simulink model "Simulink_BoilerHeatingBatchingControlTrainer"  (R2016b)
settings: Solver=VariableStepAuto  StartTime=0.0  StopTime=10000  RelTol=1e-3
libraries: simulink x28, sldrtlib x1
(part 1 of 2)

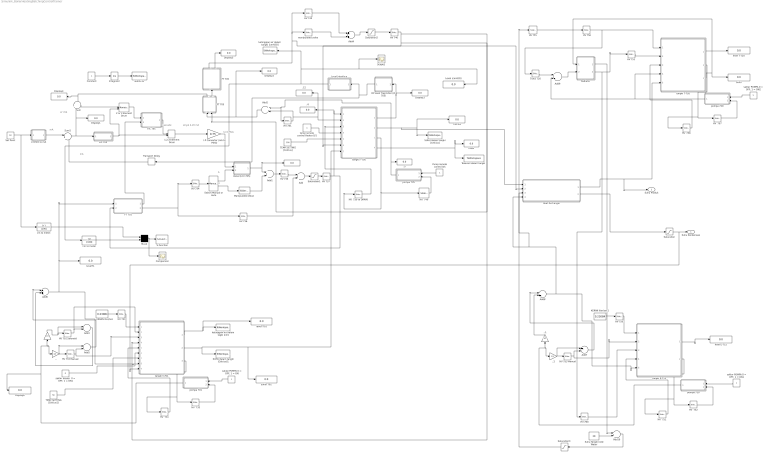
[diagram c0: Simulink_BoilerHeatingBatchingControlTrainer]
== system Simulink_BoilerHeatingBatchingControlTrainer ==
  note: Cascade
  note: 3-15 PSIG
  note: sinyal 4-20 mA
  note: mA
  note: mA
  note: A
  note: M
  note: LY 705
  ,. : Gain  RequirementInfo={} %GIDa_bc6fd614_1e62_4264_bb40_c7e61a15a363  Gain=1/2
  ,.1 : Gain  RequirementInfo={} %GIDa_cd3a2171_fe69_4d4d_90e5_3d5dc6404d7a  Gain=1/2
  .{,4..5,12} (4 alike) : Display
  .. : Gain  RequirementInfo={} %GIDa_859532f5_c8c5_4781_ad2a_2db76b1b0162  Gain=1/2
  ..1 : Gain  RequirementInfo={} %GIDa_722c5080_becd_473d_ad40_ed0b84a7ea39  Gain=1/2
  1,2,3 Element Drum : ManualSwitch  RequirementInfo={} %GIDa_e58d0757_014f_44f7_80c0_e7d97992c8d3
  2 or 3 Element Drum : ManualSwitch  RequirementInfo={} %GIDa_d69926c1_c1c0_413a_8fbd_7b981b4ad26d
  Add : Sum  RequirementInfo={} %GIDa_c8390c13_8fd0_46df_8b58_13085c3a574c
  Add1 : Sum  RequirementInfo={} %GIDa_43a3cd99_9539_4bf4_aa38_f64441418061
  Add10 : Sum
  Add2 : Sum  RequirementInfo={} %GIDa_35422669_7b0e_4bcd_b576_fa91f67b7c5f  Inputs=+-
  Add3 : Sum  RequirementInfo={} %GIDa_245dbbd9_2a0c_48cd_a41a_d83b265a6bdd  Inputs=+-
  Add4 : Sum  RequirementInfo={} %GIDa_1ca55e4e_7342_4df2_928e_79c2ac039fe9
  Add5 : Sum  RequirementInfo={} %GIDa_0dae67ae_8a33_45ca_89f9_5b09ff576389  Inputs=+-
  Add6 : Sum  RequirementInfo={} %GIDa_dee49598_737e_4bad_9513_14ba838757e0
  Add7 : Sum  RequirementInfo={} %GIDa_2ce0eeb6_1b8d_4e7c_881e_5b71408a7b6b  Inputs=+-
  Add8 : Sum  RequirementInfo={} %GIDa_35156967_a8ad_416d_ba36_a8f07401a50b
  Add9 : Sum
  Celcius : Display
  Comparison : Scope
  Constant : Constant  RequirementInfo={} %GIDa_0a77b0a1_350e_440f_9ee6_370cb4b1a8c2
  DP level Trasmitter (LT 705) : Subsystem  RequirementInfo={} %GIDa_fc1ec414_0db0_44f5_8f4f_154f58e86ad4
  Display{1..6} (6 alike) : Display
  FIC 701 : Subsystem  RequirementInfo={} %GIDa_2fdcdd1a_f8c8_4faf_bf04_b6ec306174f3
  FT 701 : Subsystem  RequirementInfo={} %GIDa_a0f6cfab_fe60_4a23_9956_c3a14955b270
  FT 705 : Subsystem  RequirementInfo={} %GIDa_2a8cb2f5_cffc_4b5e_9a3b_0ab803570460
  "HV  731 " : simulink/Math Operations/Slider Gain  low=0  gain=0  high=1
  HV  732 : simulink/Math Operations/Slider Gain  low=0  gain=1  high=1
  "HV  739 to DRAIN " : simulink/Math Operations/Slider Gain  low=0  gain=0  high=1
  "HV  740 " : simulink/Math Operations/Slider Gain  low=0  gain=1  high=1
  "HV  751 " : simulink/Math Operations/Slider Gain  low=0  gain=0  high=1
  HV  752 : simulink/Math Operations/Slider Gain  low=0  gain=1  high=1
  HV  757 : simulink/Math Operations/Slider Gain  low=0  gain=0  high=1
  HV  758 : simulink/Math Operations/Slider Gain  low=0  gain=0  high=1
  HV 701 Selenoid : simulink/Math Operations/Slider Gain  low=0  gain=0  high=1
  HV {730,735,750,756} (4 alike) : simulink/Math Operations/Slider Gain  low=0  gain=1  high=1
  HV 733 Manual : simulink/Math Operations/Slider Gain  low=0  gain=0  high=1
  "HV 734 " : simulink/Math Operations/Slider Gain  low=0  gain=1  high=1
  "HV 736 " : simulink/Math Operations/Slider Gain  low=0  gain=0  high=1
  "HV 737 " : simulink/Math Operations/Slider Gain  low=0  gain=1  high=1
  "HV 741 " : simulink/Math Operations/Slider Gain  low=0  gain=0  high=1
  HV 745 : simulink/Math Operations/Slider Gain  low=0  gain=0  high=1
  "HV 746 " : simulink/Math Operations/Slider Gain  low=0  gain=0.42086  high=1
  HV 751 : simulink/Math Operations/Slider Gain  low=0  gain=0  high=1
  HV 753 Manual : simulink/Math Operations/Slider Gain  low=0  gain=0  high=1
  "HV 755 " : simulink/Math Operations/Slider Gain  low=0  gain=1  high=1
  HV 760 : simulink/Math Operations/Slider Gain  low=0  gain=0  high=1
  Heat Exchanger : Subsystem
  I-P Converter (mA to PSIG) : Gain  RequirementInfo={} %GIDa_94b4f86c_9518_4108_a00c_4c2df90be3c9  Gain=0.75
  Integrator : Integrator  RequirementInfo={} %GIDa_4e981432_c823_455d_abdb_dc0f96a2a81a
  KERAN liter/sec : Constant  RequirementInfo={} %GIDa_cd72188c_dece_4be4_a14c_18aa689ca944  Value=0.23084
  KERAN liter/sec1 : Constant  RequirementInfo={} %GIDa_347f128a_a42e_4583_8b7f_c9f9fa14a285  Value=0.23084
  LIC 705 : Subsystem  RequirementInfo={} %GIDa_6249f34d_5a8b_41d9_ab20_0f82bded8f5b
  Level (cmH2O) : Display
  Level interface : Subsystem
  Manipulated Value : simulink/Math Operations/Slider Gain  low=0  gain=0  high=1
  Mux2 : Mux  RequirementInfo={} %GIDa_29235980_f912_414a_b16b_746e8be0c17d  Inputs=2
  PT 705 : Subsystem  RequirementInfo={} %GIDa_035bf6b7_6e08_480d_9a76_687a544ea6fb
  Pump remote control 0/1 : Constant  RequirementInfo={} %GIDa_9d76e44e_0bfb_4235_a62c_3277d40e00dd
  Radiator : Subsystem
  S-Function : S-Function  RequirementInfo={} %GIDa_3457ab31_c587_4ad5_a8ae_f74312ab7fb9  FunctionName=animtank  Parameters=1  SFunctionDeploymentMode=off  EnableBusSupport=off
  SUHU dalam tangki [Celcius] : ToWorkspace  VariableName=suhuF705  SampleTime=-1
  SUHU dalam tangki [Celcius]1 : ToWorkspace  VariableName=suhuT701  SampleTime=-1
  Saturation : Saturate  UpperLimit=5  LowerLimit=-9999999999999999999999  LinearizeAsGain=off
  Saturation1 : Saturate  RequirementInfo={} %GIDa_92280b64_3dca_498a_8f97_4b922c6ffe72  UpperLimit=1  LowerLimit=-99999999999999999999  LinearizeAsGain=off  ZeroCross=off
  Saturation2 : Saturate  RequirementInfo={} %GIDa_c6f00ae1_779b_49a9_846a_d92e31b6929e  UpperLimit=1  LowerLimit=-99999999999999999999  LinearizeAsGain=off  ZeroCross=off
  Saturation3 : Saturate  UpperLimit=28  LowerLimit=-9999999999999999  LinearizeAsGain=off
  Scope1 : Scope
  Set Point : Constant  Value=50
  Suhu : Display
  Suhu Tangki Cold Water : Constant  Value=28
  Sum : Sum  RequirementInfo={} %GIDa_2344363e_6328_49b0_a0c7_49a7caf909fe
  Sum1 : Sum  RequirementInfo={} %GIDa_c9939160_f8c3_468b_92a8_c76b635c367b  Inputs=|+-
  Switch Manual or Auto : simulink/Signal Routing/Manual Variant Sink  NumChoices=2  OverrideUsingVariant=V_1
  TEMP SETTING [Celcius] : Constant  RequirementInfo={} %GIDa_c1241bea_a72e_4e3d_bd4c_e18ce5dfffc9  Value=100
  TEMP SETTING [Celcius]1 : Constant  RequirementInfo={} %GIDa_1ee9e53c_fcbf_4bbe_a5b7_429d3d89aa33  Value=58
  TV/LV 720 : simulink/Math Operations/Slider Gain  low=0  gain=0  high=1
  "Tekanan dalam tangki " : ToWorkspace  VariableName=PressureF705  SampleTime=-1
  Transport Delay : TransportDelay
  Valve (LCV 705) : Subsystem  RequirementInfo={} %GIDa_cd02d2c4_9346_4b3f_af1b_c75ea5c89284
  cm to meter : TransferFcn  RequirementInfo={} %GIDa_bbce1113_4bf0_4329_b7d1_9b94b9680a34  Denominator=[100]
  cm to meter. : TransferFcn  RequirementInfo={} %GIDa_b4884718_8c5b_4fb0_8dff_b77bebcfc2f4  Denominator=[100]
  cmH2O to mA : Subsystem  RequirementInfo={} %GIDa_14021b81_10be_46ab_9522_3e35a22257df
  ketinggian air dalam tagki [cm] : ToWorkspace  VariableName=levelT701  SampleTime=-1
  ketinggian air dalam tangki [cmH2O] : ToWorkspace  VariableName=levelF705  SampleTime=-1
  level E-715 : Display
  level T-720 : Display
  levelT1 : Display
  levelT701 : Display
  manipulated valve : simulink/Math Operations/Slider Gain  low=0  gain=0.4  high=1
  mbar : Display
  pompa 701 : Subsystem  RequirementInfo={} %GIDa_f7b4c754_61d7_4523_a81d_5256af5e1442
  pompa 705 : Subsystem  RequirementInfo={} %GIDa_02e24820_9fe5_4fd9_b259_287392cabf84
  pompa 710 : Subsystem  RequirementInfo={} %GIDa_b40a5599_de7f_4543_949f_3323316adce9
  pompa 720 : Subsystem  RequirementInfo={} %GIDa_f39004c0_b4ae_4207_b1f8_c634ffc86dde
  "saklar heater  0 = OFF, 1 = ON1" : Constant  RequirementInfo={} %GIDa_29de96b5_5b8c_45ee_9680_99e645fe6211  Value=0
  "saklar POMPA 0 = OFF, 1 = ON" : Constant  RequirementInfo={} %GIDa_a2852ddb_fd6c_410b_b77d_b834fbe16be1
  "saklar POMPA 0 = OFF, 1 = ON1" : Constant  RequirementInfo={} %GIDa_d849ad1c_b491_4c30_8654_50d8025a813b
  "saklar POMPA 0 = OFF, 1 = ON2" : Constant  RequirementInfo={} %GIDa_87c96371_1090_42d7_9fd6_9dd4cd23a96a
  suhuT701 : Display
  tangki E-715 : Subsystem  RequirementInfo={} %GIDa_7bb4fadf_321c_4784_a602_bcf40fa0e2b0
  tangki F-705 : Subsystem  RequirementInfo={} %GIDa_ed91acdd_745b_4032_84c5_2be48a41ff32
  tangki T-701 : Subsystem  RequirementInfo={} %GIDa_4afd4461_0754_42e6_9c77_3d28637661d7
  tangki T-720 : Subsystem  RequirementInfo={} %GIDa_6bab6ea5_4044_4b9e_bbaf_a20bbf9bb028
  temp remote control Heater 0/1 : Constant  RequirementInfo={} %GIDa_5fa8f3d8_80e1_44eb_9f78_5bcca4947130
  waktu-ta' : ToWorkspace  VariableName=time  SampleTime=-1
  Suhu Kondensasi : Outport
  Suhu Produk : Outport  Port=2
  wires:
  Constant/1 -> Integrator/1
  tangki F-705/3(flow out [Liter/sec]) -> "HV  739 to DRAIN "/1, "HV  740 "/1
  "HV  739 to DRAIN "/1 -> tangki F-705/3(In6)
  "HV 736 "/1 -> Add/2
  HV 735/1 -> Add/1
  TEMP SETTING [Celcius]/1 -> tangki F-705/5(setting)
  FT 705/1(Out1) -> Display4/1, Sum/1
  FIC 701/1(Control) -> 1,2,3 Element Drum/1
  Add/1 -> Saturation1/1
  Mux2/1 -> S-Function/1, Comparison/1
  Pump remote control 0/1/1 -> pompa 705/1(saklar remote)
  Integrator/1 -> waktu-ta'/1
  FT 705/2("Out2 ") -> PT 705/1("In ")
  "HV 741 "/1 -> Add2/2, .12/1, tangki F-705/2(In2)
  "HV 734 "/1 -> Switch Manual or Auto/1
  Switch Manual or Auto/2 -> Manipulated Value/1
  Manipulated Value/1 -> Add1/2
  Add1/1 -> HV 735/1
  FT 701/2(Out2) -> "HV 734 "/1, "HV 736 "/1
  pompa 705/1(Out1) -> .5/1, Add2/1, "HV 741 "/1
  tangki F-705/4(Pressure (Pa)) -> mbar/1, "Tekanan dalam tangki "/1
  cm to meter/1 -> Mux2/2
  cm to meter./1 -> Mux2/1
  Set Point/1 -> cm to meter./1, cmH2O to mA/1(In1)
  cmH2O to mA/1(Out1) -> Sum1/1
  Switch Manual or Auto/1 -> Valve (LCV 705)/2(In2)
  I-P Converter (mA to PSIG)/1 -> Valve (LCV 705)/1(In1)
  Valve (LCV 705)/1(Out1) -> ./1, Add1/1
  LIC 705/1(Control) -> 2 or 3 Element Drum/2, 1,2,3 Element Drum/2
  temp remote control Heater 0/1/1 -> tangki F-705/4(remote on/off)
  Level interface/1(Out1) -> ketinggian air dalam tangki [cmH2O]/1, Scope1/1, Level (cmH2O)/1, cm to meter/1
  PT 705/2(Pressure Flow) -> Display5/1
  "HV  740 "/1 -> pompa 705/2(In2)
  Add6/1 -> levelT1/1, FT 701/1(In), tangki T-701/8(In7)
  Saturation2/1 -> "HV 746 "/1
  Add4/1 -> Saturation2/1
  manipulated valve/1 -> Add4/2
  HV 745/1 -> Add4/1
  "HV 746 "/1 -> tangki T-701/4(In4), FT 705/2(Valve), tangki F-705/6(In3)
  DP level Trasmitter (LT 705)/1(Out1) -> Transport Delay/1, Level interface/1(In1)
  Add2/1 -> FT 705/1(In), Display2/1
  Transport Delay/1 -> Sum1/2
  tangki F-705/1(level [cm]) -> Display3/1, DP level Trasmitter (LT 705)/1(In1)
  2 or 3 Element Drum/1 -> FIC 701/1(Set Point)
  Saturation1/1 -> "HV 737 "/1
  1,2,3 Element Drum/1 -> I-P Converter (mA to PSIG)/1
  Sum/1 -> 2 or 3 Element Drum/1
  Sum1/1 -> Display1/1, Sum/2, LIC 705/1(error)
  "HV 737 "/1 -> FT 701/2(valve), .4/1, tangki F-705/1(In1)
  FT 701/1(Out1) -> FIC 701/2(flow in)
  tangki T-701/1(level [cm]) -> ketinggian air dalam tagki [cm]/1, levelT701/1
  HV 730/1 -> tangki T-701/1(In1)
  KERAN liter/sec/1 -> HV 730/1
  pompa 701/1(Out1) -> ,./1, ../1, Display6/1
  "saklar POMPA 0 = OFF, 1 = ON"/1 -> pompa 701/1(saklar remote)
  tangki T-701/3(debit out (Liter/sec)) -> "HV  731 "/1, HV  732/1
  "HV  731 "/1 -> tangki T-701/5(In6)
  TEMP SETTING [Celcius]1/1 -> tangki T-701/7(setting)
  HV 733 Manual/1 -> tangki T-701/3(In3), Add5/2
  HV 701 Selenoid/1 -> tangki T-701/2(In2), Add3/2
  Add3/1 -> Add6/2
  Add5/1 -> Add6/1
  ../1 -> Add3/1, HV 701 Selenoid/1
  ,./1 -> Add5/1, HV 733 Manual/1
  HV  732/1 -> pompa 701/2(In2)
  "saklar heater  0 = OFF, 1 = ON1"/1 -> tangki T-701/6(remote on/off)
  Saturation/1 -> tangki T-701/9(Suhu Kondensasi), Suhu Kondensasi/1
  Heat Exchanger/1(Out1) -> tangki T-720/5(Suhu T-720), Suhu Produk/1
  Heat Exchanger/2(Out2) -> Saturation/1
  tangki F-705/2(suhu [Celcius]) -> Heat Exchanger/1(In1), Celcius/1, SUHU dalam tangki [Celcius]/1
  PT 705/1(Out1) -> Heat Exchanger/2(In2), HV 745/1, manipulated valve/1
  Add8/1 -> "HV 755 "/1, Heat Exchanger/4(In4), tangki E-715/5(In7)
  tangki T-701/2(suhu [Celcius]) -> tangki F-705/7(Suhu dari Heat Exchager), suhuT701/1, SUHU dalam tangki [Celcius]1/1
  tangki E-715/1(level [cm]) -> level E-715/1
  HV 750/1 -> tangki E-715/1(In1)
  KERAN liter/sec1/1 -> HV 750/1
  HV 760/1 -> tangki E-715/3(In4)
  pompa 710/1(Out1) -> ,.1/1, ..1/1
  "saklar POMPA 0 = OFF, 1 = ON1"/1 -> pompa 710/1(saklar remote)
  tangki E-715/2(debit out (Liter/sec)) -> "HV  751 "/1, HV  752/1
  "HV  751 "/1 -> tangki E-715/4(In6)
  HV 753 Manual/1 -> tangki E-715/2(In3), Add7/2
  ..1/1 -> Add8/2
  Add7/1 -> Add8/1
  ,.1/1 -> Add7/1, HV 753 Manual/1
  HV  752/1 -> pompa 710/2(In2)
  Radiator/2(Out2) -> HV 760/1, HV 751/1
  tangki T-720/1(level [cm]) -> level T-720/1
  "HV 755 "/1 -> HV 756/1
  "saklar POMPA 0 = OFF, 1 = ON2"/1 -> pompa 720/1(saklar remote)
  tangki T-720/2(debit out (Liter/sec)) -> HV  758/1, HV  757/1
  HV  758/1 -> tangki T-720/3(In6)
  HV  757/1 -> pompa 720/2(In2)
  HV 756/1 -> TV/LV 720/1, tangki T-720/1(In3)
  HV 751/1 -> tangki T-720/2(In4)
  TV/LV 720/1 -> Add9/1
  Add9/1 -> Radiator/2(In2)
  pompa 720/1(Out1) -> tangki T-720/4(In7), Add9/2
  tangki T-720/3(Suhu. T-720) -> Radiator/1(In1), Suhu/1
  Suhu Tangki Cold Water/1 -> Add10/2
  Add10/1 -> Saturation3/1
  Radiator/1(Out1) -> Add10/1
  Saturation3/1 -> Heat Exchanger/3(In3)

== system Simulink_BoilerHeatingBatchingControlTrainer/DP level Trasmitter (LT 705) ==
  note: P
  note: Tekanan hidrostatis P = p g h dimana P = Tekanan hidrostatis (N/m^2) g = percepatan gravitasi (m/s^2) p = massa jenis air (kg/m^3) h = level fluida
  note: mA
  In1 : Inport  RequirementInfo={} %GIDa_65631801_4d77_4024_98a1_8120f602e0b4
  Bias : Bias  RequirementInfo={} %GIDa_f33fa9ee_ffc2_4756_a0a9_dfedda8f7d97  Bias=4
  DP Level Transmitter Transfer Function : TransferFcn  RequirementInfo={} %GIDa_e8153e25_1b53_45ed_b90f_907755ff59fb  Numerator=[0.0016]  Denominator=[2 1]
  Saturation : Saturate  RequirementInfo={} %GIDa_8eb5f573_8386_419d_8ff5_e8c857dd8568  UpperLimit=100  LowerLimit=0
  cm to meter : TransferFcn  RequirementInfo={} %GIDa_c943a8fa_65e2_4f5a_9149_849483c8273c  Denominator=[100]
  "massa jenis air (kg/m^3) " : Gain  Gain=1000
  percepatan gravitasi (m/s^2) : Gain  Gain=10
  Out1 : Outport  RequirementInfo={} %GIDa_2639bf9d_f08e_47f0_818f_697f90294355
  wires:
  Bias/1 -> Out1/1
  DP Level Transmitter Transfer Function/1 -> Bias/1
  Saturation/1 -> cm to meter/1
  cm to meter/1 -> percepatan gravitasi (m/s^2)/1
  percepatan gravitasi (m/s^2)/1 -> "massa jenis air (kg/m^3) "/1
  "massa jenis air (kg/m^3) "/1 -> DP Level Transmitter Transfer Function/1
  In1/1 -> Saturation/1

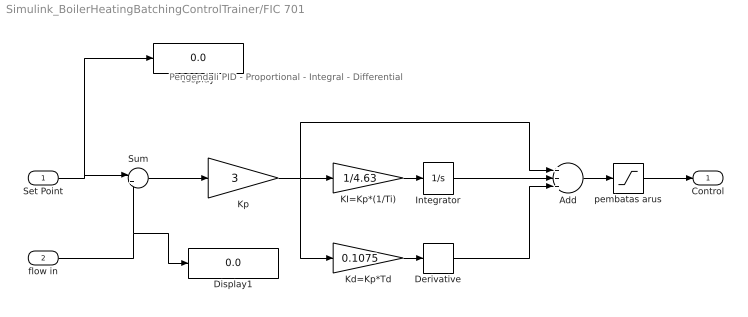
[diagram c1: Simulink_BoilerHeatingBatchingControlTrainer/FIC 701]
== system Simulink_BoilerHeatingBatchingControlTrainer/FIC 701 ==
  note: Pengendali PID - Proportional - Integral - Differential
  Set Point : Inport  RequirementInfo={} %GIDa_9f8afcc0_bd88_4eb8_a97b_6ecc268b5e18
  flow in : Inport  RequirementInfo={} %GIDa_c4b25152_8ee0_44cb_adf6_79b81e7e58c5  Port=2
  Add : Sum  RequirementInfo={} %GIDa_17127419_3f62_415e_aa71_fe9c3b791bdc  Inputs=+++
  Derivative : Derivative  RequirementInfo={} %GIDa_3cb770cc_eb01_4b5e_b710_f54f731fb878
  Display : Display
  Display1 : Display
  Integrator : Integrator  RequirementInfo={} %GIDa_572a1376_a49e_41ff_a672_043c82c3386a  WrappedStateUpperValue=1  WrappedStateLowerValue=0  AbsoluteTolerance=0.000001
  KI=Kp*(1/Ti) : Gain  RequirementInfo={} %GIDa_284b2896_22a0_4b96_b62d_05058d48bb7a  Gain=1/4.63
  Kd=Kp*Td : Gain  RequirementInfo={} %GIDa_d6db21fb_5bd6_40ce_b4f8_d65536af4805  Gain=0.1075
  Kp : Gain  RequirementInfo={} %GIDa_c2ca3795_47e7_440f_9f70_1098747fe6dc  Gain=3
  Sum : Sum  RequirementInfo={} %GIDa_06ad238c_f061_48da_9d84_753d56ea98e4  Inputs=|+-
  pembatas arus : Saturate  RequirementInfo={} %GIDa_9162f0eb_568f_4d07_b800_862de9305c7a  UpperLimit=20  LowerLimit=4  LinearizeAsGain=off  ZeroCross=off
  Control : Outport  RequirementInfo={} %GIDa_3827570e_3741_4a35_99cf_65f942aa179c
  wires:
  Set Point/1 -> Display/1, Sum/1
  Derivative/1 -> Add/3
  Kd=Kp*Td/1 -> Derivative/1
  KI=Kp*(1/Ti)/1 -> Integrator/1
  Integrator/1 -> Add/2
  Sum/1 -> Kp/1
  Kp/1 -> Add/1, KI=Kp*(1/Ti)/1, Kd=Kp*Td/1
  flow in/1 -> Display1/1, Sum/2
  Add/1 -> pembatas arus/1
  pembatas arus/1 -> Control/1

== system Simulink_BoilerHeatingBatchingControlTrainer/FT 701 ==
  note: mA
  In : Inport  RequirementInfo={} %GIDa_75747b92_ec31_4a77_855f_7f8408e9e0c8
  valve : Inport  RequirementInfo={} %GIDa_9b77dd24_a13f_4a54_955e_505fd564a108  Port=2
  Display : Display
  Display1 : Display
  Display2 : Display
  Product : Product  RequirementInfo={} %GIDa_2bc26cfb_ca2f_49ad_bdfd_cca0e444ba62
  Vorterx Flowmeter Transmitter : Subsystem  RequirementInfo={} %GIDa_7df4c895_af51_4c28_970e_91438a065f96
  Out1 : Outport  RequirementInfo={} %GIDa_25f778d7_c91a_416d_97c4_224487e145cd
  Out2 : Outport  RequirementInfo={} %GIDa_5f09f169_334b_4675_8f30_9d38aae03e30  Port=2
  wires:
  valve/1 -> Product/1
  In/1 -> Display1/1, Out2/1, Product/2
  Vorterx Flowmeter Transmitter/1(Out1) -> Out1/1, Display/1
  Product/1 -> Display2/1, Vorterx Flowmeter Transmitter/1(In1)

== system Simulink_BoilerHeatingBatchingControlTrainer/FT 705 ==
  note: mA
  In : Inport  RequirementInfo={} %GIDa_c1c88e7e_e9c8_46ea_a939_2ca83d4af817
  Valve : Inport  RequirementInfo={} %GIDa_d8e79c6c_2e12_4639_b81a_cc08f1b3ff74  Port=2
  Display2 : Display
  Orifice D/P Transmitter : Subsystem  RequirementInfo={} %GIDa_d9d61335_7f9e_4fb6_b4bd_8fb0e7619f15
  Product : Product
  mA : Display
  Out1 : Outport  RequirementInfo={} %GIDa_be75002b_0f28_414e_b45f_00a185a07d57
  "Out2 " : Outport  RequirementInfo={} %GIDa_194db342_4ec6_46f7_bc90_f43f5a113e2a  Port=2
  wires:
  In/1 -> Product/2, Display2/1, "Out2 "/1
  Orifice D/P Transmitter/1(Out1) -> mA/1, Out1/1
  Valve/1 -> Product/1
  Product/1 -> Orifice D/P Transmitter/1(In1)

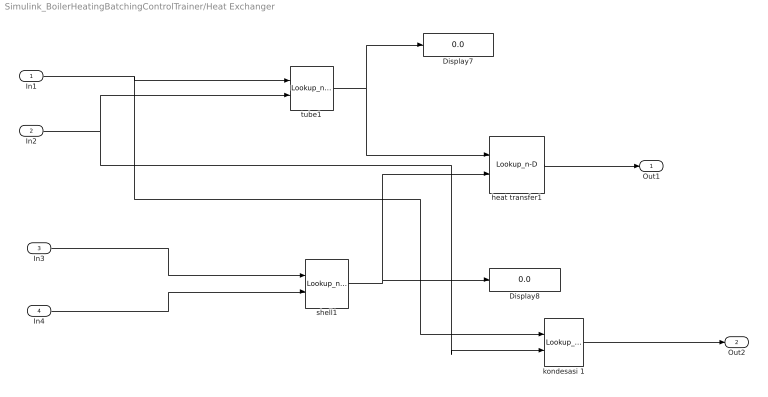
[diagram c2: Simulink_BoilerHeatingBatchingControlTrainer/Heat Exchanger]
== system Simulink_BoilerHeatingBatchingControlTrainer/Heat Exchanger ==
  In1 : Inport
  In2 : Inport  Port=2
  In3 : Inport  Port=3
  In4 : Inport  Port=4
  Display7 : Display
  Display8 : Display
  heat transfer1 : Lookup_n-D  BreakpointsForDimension1=[20,25,30]  BreakpointsForDimension2=[22,23,28,32,34,36,38,39,40,41,42,43,44,45,46,47,48,49,50,51,52,53,54,55,56,57,58,59,60,61,62]  Table=reshape([28,30,33,29,31,34,29,31,34,30,32,35,31,33,36,31,34,36,31,34,37,32,34,38,32,35,39,33,35,40,33,36,40,34,36,41,35,37,41,35,37,42,36,38,43,37,38,44,37,39,45,37,39,45,38,40,45,38,40,46,38,41,47,38,41,48,38,42,49,38,42,50,38,43,50,39,43,51,39,44,52,39,44,52,39,45,53,39,46,54,39,47,55],3,31)  InternalRulePriority=Speed  RndMeth=Simplest
  kondesasi 1 : Lookup_n-D  BreakpointsForDimension1=[37.7,38.1,38.2,38.4,38.5,38.6,38.7,38.9,40,40.1,40.2,40.3,40.4,40.5,40.6,40.7,40.8,40.9,41,41.1,41.2,41.3,41.4,41.5,41.6,41.7,41.8,41.9,42,42.1,42.2,42.3,42.4,42.5,42.6,42.7,42.8]  BreakpointsForDimension2=[21,22,27,28,32,34,35,37,38,39,40,41,42,43,45,46,48,49,50,51,52,53,54,55,56,57,58,59,60,61,62,63,64,65,66,67,68]  Table=reshape([28,0,0,0,0,0,0,0,0,0,0,0,0,0,0,0,0,0,0,0,0,0,0,0,0,0,0,0,0,0,0,0,0,0,0,0,0,0,28,0,0,0,0,0,0,0,0,0,0,0,0,0,0,0,0,0,0,0,0,0,0,0,0,0,0,0,0,0,0,0,0,0,0,0,0,0,28,0,0,0,0,0,0,0,0,0,0,0,0,0,0,0,0,0,0,0,0,0,0,0,0,0,0,0,0,0,0,0,0,0,0,0,0,0,28,0,0,0,0,0,0,0,0,0,0,0,0,0,0,0,0,0,0,0,0,0,0,0,0,0,0,0,0,0,0,0,0,0,0,0,0,0,28,0,0,0,0,0,0,0,0,0,0,0,0,0,0,0,0,0,0,0,0,0,0,0,0,0,0,0,0,0,0,0,0,0,0,0,0,0,28,0,0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  InternalRulePriority=Speed  RndMeth=Simplest
  shell1 : Lookup_n-D  BreakpointsForDimension1=[22,23,24,25,26,27,28,29,30,31,32,33,34,35,36,37,38,39,40,41,42,43,44,45,46,47,48,49,50,51]  BreakpointsForDimension2=[20,30,40]  Table=reshape([20,20,20,20,20,20,20,20,20,20,20,20,20,20,20,20,20,20,20,20,20,20,20,20,20,20,20,20,20,20,30,30,30,30,30,30,30,30,30,30,30,30,30,30,30,30,30,30,30,30,30,30,30,30,30,30,30,30,30,30,40,40,40,40,40,40,40,40,40,40,40,40,40,40,40,40,40,40,40,40,40,40,40,40,40,40,40,40,40,40],30,3)  InternalRulePriority=Speed  RndMeth=Simplest
  tube1 : Lookup_n-D  BreakpointsForDimension1=[37.7,38.2,38.6,39.1,39.6,40,40.2,40.4,40.9,41,41.1,41.2,41.3,41.4,41.5,41.6,41.7,41.8]  BreakpointsForDimension2=[50.5,60.5,65.5]  Table=reshape([20,20,24,24,25,26,26,27,28,29,29,30,31,32,32,33,34,34,21,23,23,23,25,26,28,29,29,30,31,33,35,35,35,36,36,37,22,28,28,32,34,36,38,39,39,40,41,43,44,45,46,47,48,48],18,3)  InternalRulePriority=Speed  RndMeth=Simplest
  Out1 : Outport
  Out2 : Outport  Port=2
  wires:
  In3/1 -> shell1/1
  In2/1 -> kondesasi 1/2, tube1/2
  In4/1 -> shell1/2
  tube1/1 -> Display7/1, heat transfer1/1
  heat transfer1/1 -> Out1/1
  In1/1 -> kondesasi 1/1, tube1/1
  shell1/1 -> heat transfer1/2, Display8/1
  kondesasi 1/1 -> Out2/1

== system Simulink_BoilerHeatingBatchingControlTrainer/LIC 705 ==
  error : Inport  RequirementInfo={} %GIDa_4ad8dbd3_b741_4310_bc15_0ee86257d960
  " Ki = Kp*(1/Ti)" : Gain  RequirementInfo={} %GIDa_d188301b_612d_46a0_803a_a337453cbc52  Gain=1/4.91
  Add : Sum  RequirementInfo={} %GIDa_fa0f6e8b_4c88_4899_9bc4_8c8ab8ca893d  Inputs=+++
  Derivative : Derivative  RequirementInfo={} %GIDa_f304c9a2_4ff9_440e_b3ce_e9561c6185e4
  Integrator : Integrator  RequirementInfo={} %GIDa_c4329437_8175_4879_a6b4_168e5c6bf409  WrappedStateUpperValue=1  WrappedStateLowerValue=0  AbsoluteTolerance=0.000001
  Kd= Kp*Td : Gain  RequirementInfo={} %GIDa_640666a3_b2f3_48e1_bd73_968c22c8354e  Gain=1.2275
  "Kp " : Gain  RequirementInfo={} %GIDa_1055eada_0cd8_4ff8_aa51_8a880045bfc6  Gain=60
  pembatas arus : Saturate  RequirementInfo={} %GIDa_d69760b3_5244_44c4_b0bd_ec108afab32d  UpperLimit=20  LowerLimit=4  LinearizeAsGain=off  ZeroCross=off
  Control : Outport  RequirementInfo={} %GIDa_8e66f68e_100f_429d_86da_8278e91e347b
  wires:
  Derivative/1 -> Add/3
  Kd= Kp*Td/1 -> Derivative/1
  " Ki = Kp*(1/Ti)"/1 -> Integrator/1
  Integrator/1 -> Add/2
  error/1 -> "Kp "/1
  "Kp "/1 -> Add/1, " Ki = Kp*(1/Ti)"/1, Kd= Kp*Td/1
  Add/1 -> pembatas arus/1
  pembatas arus/1 -> Control/1

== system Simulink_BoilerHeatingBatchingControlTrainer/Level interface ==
  In1 : Inport
  Bias : Bias  RequirementInfo={} %GIDa_3123f81d_955c_43e4_aad9_2af6c68f688e  Bias=-4
  Transfer Fcn : TransferFcn  Denominator=[0.16]
  Out1 : Outport
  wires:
  In1/1 -> Bias/1
  Transfer Fcn/1 -> Out1/1
  Bias/1 -> Transfer Fcn/1

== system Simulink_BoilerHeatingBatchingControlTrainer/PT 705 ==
  note: L/s
  note: mA
  "In " : Inport  RequirementInfo={} %GIDa_b404bdbe_38c2_4836_bb6e_17a2e0964302
  Bias : Bias  RequirementInfo={} %GIDa_acb53d2c_ce93_42e8_839c_39408c01fed6  Bias=4
  Display : Display
  "Pressure Transmitter " : TransferFcn  RequirementInfo={} %GIDa_709c34dd_f5b6_489f_a20b_d45708b41fbf  Numerator=[16]  Denominator=[2 1]
  Real-Time Synchronization : sldrtlib/Real-Time Synchronization  SampleTime=1  MaxMissedTicks=10  ShowMissedTicks=off  YieldWhenWaiting=off
  pressure interface : Lookup_n-D  NumberOfTableDimensions=1  BreakpointsForDimension1=[4,5,6,7,8,9,10,11,12,13,14,15,16,17,18,19,20]  Table=[0,1.875,3.75,5.625,7.5,9.375,11.25,13.125,15,16.875,18.75,20.625,22.5,24.375,26.25,28.125,30]  InternalRulePriority=Speed  RndMeth=Simplest
  Out1 : Outport  RequirementInfo={} %GIDa_bc94333d_35a0_4279_8634_c0e161b25d4f
  Pressure Flow : Outport  RequirementInfo={} %GIDa_c9181890_1c3f_4b0e_acd2_4f933bde059a  Port=2
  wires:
  "Pressure Transmitter "/1 -> Bias/1
  "In "/1 -> "Pressure Transmitter "/1, Out1/1
  Bias/1 -> pressure interface/1
  pressure interface/1 -> Pressure Flow/1, Display/1

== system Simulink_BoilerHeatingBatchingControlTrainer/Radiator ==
  In1 : Inport
  In2 : Inport  Port=2
  Radiator : Saturate  UpperLimit=28  LowerLimit=-999999999999999  LinearizeAsGain=off
  Out1 : Outport
  Out2 : Outport  Port=2
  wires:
  Radiator/1 -> Out1/1
  In1/1 -> Radiator/1
  In2/1 -> Out2/1

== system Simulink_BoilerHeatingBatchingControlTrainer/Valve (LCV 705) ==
  In1 : Inport  RequirementInfo={} %GIDa_7b2dc152_e439_464f_8419_29272025728c
  In2 : Inport  RequirementInfo={} %GIDa_0b06d359_31a0_43fa_b53a_8e78cc30c310  Port=2
  Display1 : Display
  Display2 : Display
  Display3 : Display
  Product : Product  RequirementInfo={} %GIDa_cfd4cfaf_2ec1_4d56_9dbc_252fb7013167
  Tekanan ke posisi katup : Lookup_n-D  RequirementInfo={} %GIDa_750e307a_8434_4b28_949b_0dd7ad9853c3  NumberOfTableDimensions=1  BreakpointsForDimension1=single([3,4,5,6,7,8,9,10,11,12,13,14,15]);  Table=single([0,0.08333333,0.16666666,0.25,0.33333333,0.41666666,0.5,0.58333333,0.66666666,0.75,0.83333333,0.91666666,1]);  InternalRulePriority=Speed  RndMeth=Simplest
  Out1 : Outport  RequirementInfo={} %GIDa_bd3560f0_087e_4b05_89d3_bdddfa2d4299
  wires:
  In2/1 -> Display1/1, Product/2
  Product/1 -> Out1/1
  In1/1 -> Display3/1, Display2/1, Tekanan ke posisi katup/1
  Tekanan ke posisi katup/1 -> Product/1

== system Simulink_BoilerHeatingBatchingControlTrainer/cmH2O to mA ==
  note: mA
  In1 : Inport  RequirementInfo={} %GIDa_33a28457_7c39_49b8_ba63_a88f18a37ba4
  Bias : Bias  RequirementInfo={} %GIDa_611608c1_10b7_40c9_8d0c_beb05ed1aeb9  Bias=4
  Gain : Gain  RequirementInfo={} %GIDa_bb1fd363_18ed_43c3_8ed0_c05233bcf6f1  Gain=0.16
  Out1 : Outport  RequirementInfo={} %GIDa_2419383b_7eb2_428d_800f_91797161b840
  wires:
  In1/1 -> Gain/1
  Gain/1 -> Bias/1
  Bias/1 -> Out1/1

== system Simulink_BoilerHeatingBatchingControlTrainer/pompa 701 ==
  saklar remote : Inport  RequirementInfo={} %GIDa_8dad9eb6_70c7_456e_a7c6_6662ff69968b
  In2 : Inport  RequirementInfo={} %GIDa_a95ccdaa_a920_4508_8bcf_75599c23e4af  Port=2
  Kapasitas Maksimum Pompa 60 LPM : Saturate  RequirementInfo={} %GIDa_2e1f510a_eb6b_4fc5_a27b_02ce6d2dd788  UpperLimit=1  LowerLimit=0  LinearizeAsGain=off  ZeroCross=off
  Product1 : Product  RequirementInfo={} %GIDa_9b477e04_6d92_4cac_b2e0_2b160a33d296
  Out1 : Outport  RequirementInfo={} %GIDa_fa67a272_03b0_4a34_8979_9aa4b7efb4ff
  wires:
  Kapasitas Maksimum Pompa 60 LPM/1 -> Out1/1
  Product1/1 -> Kapasitas Maksimum Pompa 60 LPM/1
  In2/1 -> Product1/2
  saklar remote/1 -> Product1/1

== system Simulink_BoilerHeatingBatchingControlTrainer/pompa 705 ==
  saklar remote : Inport  RequirementInfo={} %GIDa_0ba5ae8b_98b3_4e05_a5d7_0cde85049c6c
  In2 : Inport  RequirementInfo={} %GIDa_ac9619e0_261e_4785_ac11_461246701d2a  Port=2
  Kapasitas Maksimum Pompa 60 LPM : Saturate  RequirementInfo={} %GIDa_4610b2d7_eb4d_498c_aff6_13911aefd67b  UpperLimit=1  LowerLimit=-9999999999999999999999999999999999999999  LinearizeAsGain=off  ZeroCross=off
  Product : Product  RequirementInfo={} %GIDa_8c8a7048_9af8_4b83_9be8_730163159390
  Out1 : Outport  RequirementInfo={} %GIDa_0115c574_83f2_417a_953f_6eabdef47cb4
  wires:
  Product/1 -> Kapasitas Maksimum Pompa 60 LPM/1
  In2/1 -> Product/2
  saklar remote/1 -> Product/1
  Kapasitas Maksimum Pompa 60 LPM/1 -> Out1/1

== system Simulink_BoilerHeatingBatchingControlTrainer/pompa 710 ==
  saklar remote : Inport  RequirementInfo={} %GIDa_3a548eaf_271a_4d24_9cac_f376dc129dbc
  In2 : Inport  RequirementInfo={} %GIDa_d979bf60_b785_4625_9f08_0fdc506618a3  Port=2
  Kapasitas Maksimum Pompa 60 LPM : Saturate  RequirementInfo={} %GIDa_dd4edcb4_8b20_40a8_83a9_eeceb563408c  UpperLimit=1  LowerLimit=0  LinearizeAsGain=off  ZeroCross=off
  Product1 : Product  RequirementInfo={} %GIDa_001e17ff_f0f7_4fef_8aae_80dc789a0343
  Out1 : Outport  RequirementInfo={} %GIDa_8e3c72c1_9320_4c24_becd_27adaae7b93e
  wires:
  Kapasitas Maksimum Pompa 60 LPM/1 -> Out1/1
  Product1/1 -> Kapasitas Maksimum Pompa 60 LPM/1
  In2/1 -> Product1/2
  saklar remote/1 -> Product1/1

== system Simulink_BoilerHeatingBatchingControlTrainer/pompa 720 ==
  saklar remote : Inport  RequirementInfo={} %GIDa_55aaf99b_e2ba_4c78_a863_475a62198023
  In2 : Inport  RequirementInfo={} %GIDa_f66ebb62_d1e0_47bd_ba71_5ce329b7dee3  Port=2
  Kapasitas Maksimum Pompa 60 LPM : Saturate  RequirementInfo={} %GIDa_b016e3be_a712_4537_8610_2567f4222366  UpperLimit=1  LowerLimit=0  LinearizeAsGain=off  ZeroCross=off
  Product1 : Product  RequirementInfo={} %GIDa_b2900b07_4522_4fce_ad64_90e57baff023
  Out1 : Outport  RequirementInfo={} %GIDa_5adfb327_aceb_4cdf_8519_1afbc8977a0d
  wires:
  Kapasitas Maksimum Pompa 60 LPM/1 -> Out1/1
  Product1/1 -> Kapasitas Maksimum Pompa 60 LPM/1
  In2/1 -> Product1/2
  saklar remote/1 -> Product1/1

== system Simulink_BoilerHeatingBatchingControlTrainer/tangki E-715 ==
  In1 : Inport  RequirementInfo={} %GIDa_01cf6b6d_5f74_4ea7_8550_3b0a6498cf1a
  In3 : Inport  RequirementInfo={} %GIDa_eb169c58_ee02_47a3_b469_912cfe21415a  Port=2
  In4 : Inport  RequirementInfo={} %GIDa_dbfb1a93_13a3_43dd_a886_2101b7eb0bce  Port=3
  In6 : Inport  RequirementInfo={} %GIDa_18f12a20_9ddd_4717_adff_54757da773b2  Port=4
  In7 : Inport  RequirementInfo={} %GIDa_6b6feda6_a893_4c57_b7ed_f314fe19c545  Port=5
  Penghitung Level : Subsystem  RequirementInfo={} %GIDa_ccf60bd3_ca15_4e20_9e59_2334190f12cf
  level [cm] : Outport  RequirementInfo={} %GIDa_9ad3bea9_4d8c_4605_9731_3567490b3534
  debit out (Liter/sec) : Outport  RequirementInfo={} %GIDa_13eb8001_fe40_43ad_8a6c_72aee9ea9063  Port=2
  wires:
  In1/1 -> Penghitung Level/1(dari keran via HV-730)
  In3/1 -> Penghitung Level/2(Dari Pompa lewat HV-733)
  In6/1 -> Penghitung Level/4(Drain)
  In7/1 -> Penghitung Level/5(HV 752 ke Pompa)
  Penghitung Level/2(debit out (Liter/sec)) -> debit out (Liter/sec)/1
  Penghitung Level/1(level [cm]) -> level [cm]/1
  In4/1 -> Penghitung Level/3(Dari Heat-Exc  lewat HV-746)

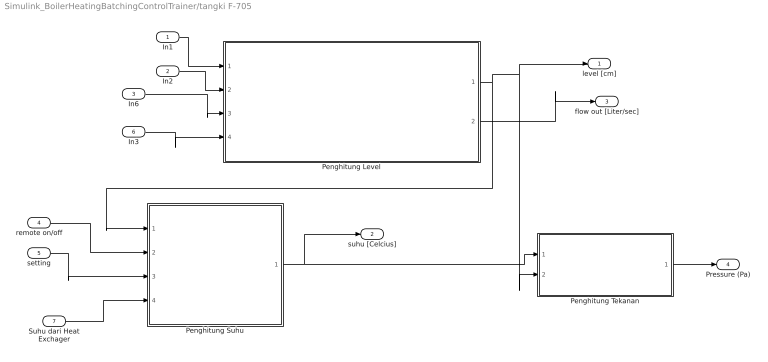
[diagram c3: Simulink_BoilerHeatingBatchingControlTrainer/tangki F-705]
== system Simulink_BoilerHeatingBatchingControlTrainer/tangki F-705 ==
  In1 : Inport  RequirementInfo={} %GIDa_bbe9b501_074f_46b1_b93a_4926bcfff15a
  In2 : Inport  RequirementInfo={} %GIDa_476b6e3e_4b05_424d_870e_804995eb0ad5  Port=2
  In6 : Inport  RequirementInfo={} %GIDa_b3e32092_b233_43e8_9931_93f01f0608d9  Port=3
  remote on/off : Inport  RequirementInfo={} %GIDa_748b98f4_ec3c_4c94_b6a6_9edf1693d771  Port=4
  setting : Inport  RequirementInfo={} %GIDa_43adf472_c096_448e_bd76_e75b64be642d  Port=5
  In3 : Inport  RequirementInfo={} %GIDa_88629ef3_09d7_4f69_aac9_861778db5afe  Port=6
  Suhu dari Heat Exchager : Inport  Port=7
  Penghitung Level : Subsystem  RequirementInfo={} %GIDa_213d0408_c3df_4d72_b83e_cee0165b2c92
  Penghitung Suhu : Subsystem  RequirementInfo={} %GIDa_392d8b63_2ebe_4767_b747_4380ea404327
  Penghitung Tekanan : Subsystem  RequirementInfo={} %GIDa_d756253b_cf02_454d_a8d9_0d7f6754dfd7
  level [cm] : Outport  RequirementInfo={} %GIDa_d3a3c32d_9bc0_43d9_896f_06108a635287
  suhu [Celcius] : Outport  RequirementInfo={} %GIDa_cc96a464_973f_4964_a9a3_9f6366ca9808  Port=2
  flow out [Liter/sec] : Outport  RequirementInfo={} %GIDa_f4789da4_0fae_4e25_8791_cc2e6c59cf84  Port=3
  Pressure (Pa) : Outport  RequirementInfo={} %GIDa_10a270c9_afdd_41d1_9189_68d0988d49a2  Port=4
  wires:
  Penghitung Suhu/1(suhu) -> suhu [Celcius]/1, Penghitung Tekanan/1(Suhu)
  In2/1 -> Penghitung Level/2(Dari Pompa lewat HV-741)
  In6/1 -> Penghitung Level/3(Drain)
  Penghitung Level/1(level [cmH2O]) -> level [cm]/1, Penghitung Tekanan/2(Level), Penghitung Suhu/1(level[cm])
  remote on/off/1 -> Penghitung Suhu/2(Remote Heater)
  In1/1 -> Penghitung Level/1(dari T-701)
  In3/1 -> Penghitung Level/4(Pompa 705)
  Penghitung Level/2(debit out (Liter/sec)) -> flow out [Liter/sec]/1
  setting/1 -> Penghitung Suhu/3(Set Point)
  Penghitung Tekanan/1(Pressure tangki (mbar)) -> Pressure (Pa)/1
  Suhu dari Heat Exchager/1 -> Penghitung Suhu/4(Suhu dari T-701)

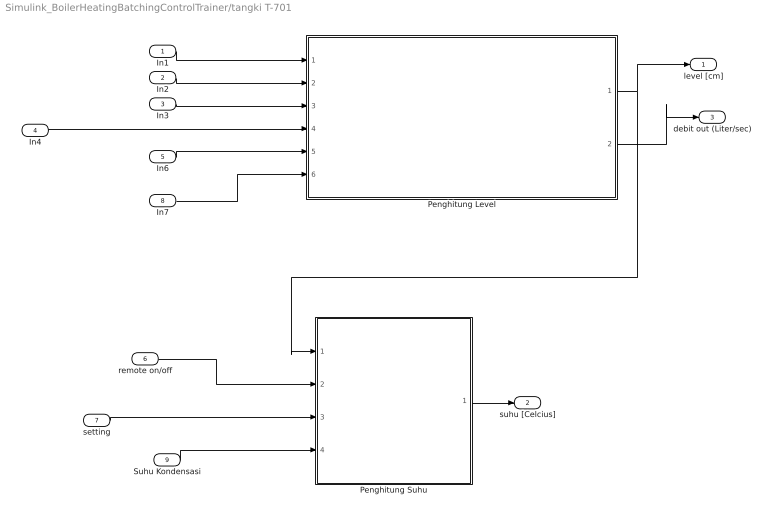
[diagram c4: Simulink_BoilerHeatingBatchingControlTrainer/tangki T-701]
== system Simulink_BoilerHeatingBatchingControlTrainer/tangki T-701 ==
  In1 : Inport  RequirementInfo={} %GIDa_462cf91c_a6d6_4f55_ba2e_56d032c13537
  In2 : Inport  RequirementInfo={} %GIDa_cc7f89db_d13c_416f_93a3_a25f142d2280  Port=2
  In3 : Inport  RequirementInfo={} %GIDa_fbe3b955_bbae_4fcb_8e42_3fb557e071db  Port=3
  In4 : Inport  RequirementInfo={} %GIDa_3e8a477f_1f31_4bd8_a79b_dc89b8a0164b  Port=4
  In6 : Inport  RequirementInfo={} %GIDa_b052aff6_590e_4db8_8c01_665342705f88  Port=5
  remote on/off : Inport  RequirementInfo={} %GIDa_349615af_c891_4330_a3fd_cabcb3723c3e  Port=6
  setting : Inport  RequirementInfo={} %GIDa_850bc7d7_cfa0_4368_9d21_40253df414b8  Port=7
  In7 : Inport  RequirementInfo={} %GIDa_5d989dae_5392_4bd8_a4d5_28ddd9a72122  Port=8
  Suhu Kondensasi : Inport  Port=9
  Penghitung Level : Subsystem  RequirementInfo={} %GIDa_447f6a26_fad7_4fc0_b6cd_e5919a574315
  Penghitung Suhu : Subsystem  RequirementInfo={} %GIDa_d60ce84b_2dd1_4b0c_8538_50bc4ab19d54
  level [cm] : Outport  RequirementInfo={} %GIDa_6b8b1b91_9612_4fd4_9cb2_82b92b8bf916
  suhu [Celcius] : Outport  RequirementInfo={} %GIDa_5ebb4fc4_dbd1_4951_9a8c_6ce364adce9e  Port=2
  debit out (Liter/sec) : Outport  RequirementInfo={} %GIDa_e55150ae_ae4a_4d03_8e62_1f7024a1532a  Port=3
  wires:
  In1/1 -> Penghitung Level/1(dari keran via HV-730)
  In2/1 -> Penghitung Level/2(Dari Pompa lewat HV-701)
  In3/1 -> Penghitung Level/3(Dari Pompa lewat HV-733)
  In6/1 -> Penghitung Level/5(Drain)
  In7/1 -> Penghitung Level/6(HV 732 ke Pompa)
  Penghitung Level/2(debit out (Liter/sec)) -> debit out (Liter/sec)/1
  Penghitung Level/1(level [cm]) -> level [cm]/1, Penghitung Suhu/1(level[cm])
  Penghitung Suhu/1(suhu) -> suhu [Celcius]/1
  remote on/off/1 -> Penghitung Suhu/2(Remote Heater)
  In4/1 -> Penghitung Level/4(Dari  lewat HV-746)
  setting/1 -> Penghitung Suhu/3(Set Point)
  Suhu Kondensasi/1 -> Penghitung Suhu/4(suhu kondensasi)

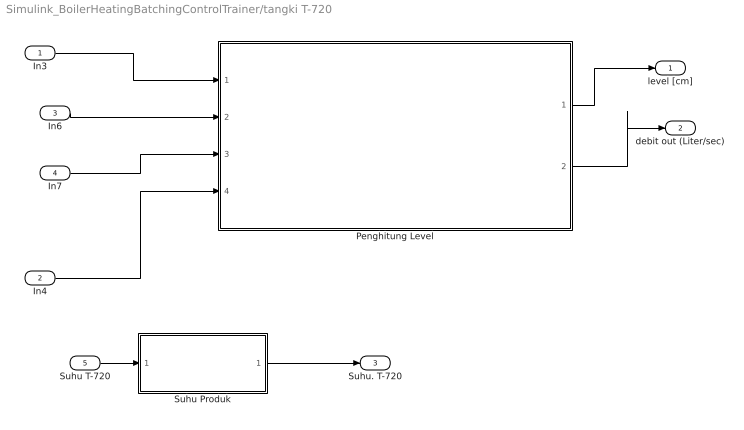
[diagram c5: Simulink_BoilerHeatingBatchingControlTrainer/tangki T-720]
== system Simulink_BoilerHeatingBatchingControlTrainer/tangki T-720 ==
  In3 : Inport  RequirementInfo={} %GIDa_f03683ba_3185_4787_886a_f180c75bcf62
  In4 : Inport  RequirementInfo={} %GIDa_9f5bc4f7_6184_435f_9b74_dfd585403fda  Port=2
  In6 : Inport  RequirementInfo={} %GIDa_fa2be3ad_23db_4b65_b36f_43777d4c8234  Port=3
  In7 : Inport  RequirementInfo={} %GIDa_fb7fd1a2_a6b1_423e_a588_95ecd29e0bcd  Port=4
  Suhu T-720 : Inport  Port=5
  Penghitung Level : Subsystem  RequirementInfo={} %GIDa_b3b2ac41_6440_4e62_bc67_a9b086fd9137
  Suhu Produk : Subsystem
  level [cm] : Outport  RequirementInfo={} %GIDa_a095bdbb_dc4e_4360_92b8_51508d621331
  debit out (Liter/sec) : Outport  RequirementInfo={} %GIDa_b396ae19_2cc8_40e3_8640_cc659762e31b  Port=2
  Suhu. T-720 : Outport  Port=3
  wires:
  Penghitung Level/2(debit out (Liter/sec)) -> debit out (Liter/sec)/1
  Penghitung Level/1(level [cm]) -> level [cm]/1
  Suhu T-720/1 -> Suhu Produk/1(Suhu T-720)
  Suhu Produk/1(Suhu. T-720) -> Suhu. T-720/1
  In3/1 -> Penghitung Level/1(Dari Heat-Exc  lewat HV-756)
  In4/1 -> Penghitung Level/4(Pompa ke HV 751)
  In6/1 -> Penghitung Level/2(Drain)
  In7/1 -> Penghitung Level/3(HV 757 ke Pompa)

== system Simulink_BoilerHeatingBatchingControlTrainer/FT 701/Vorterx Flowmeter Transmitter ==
  note: mA
  In1 : Inport  RequirementInfo={} %GIDa_6e975a63_666b_4a0b_ad79_cdd211a48e0d
  Bias : Bias  RequirementInfo={} %GIDa_b0253cc1_8a41_4a45_976d_494b91ace727  Bias=4
  Vortex Flowmeter Transmitter Transfer Function : TransferFcn  RequirementInfo={} %GIDa_7d5008a2_f2ad_4b8f_9af3_0560dd37fa3c  Numerator=[16]  Denominator=[4 1]
  Out1 : Outport  RequirementInfo={} %GIDa_538867de_a97a_4475_819d_7f2d4ad8eeff
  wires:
  Vortex Flowmeter Transmitter Transfer Function/1 -> Bias/1
  Bias/1 -> Out1/1
  In1/1 -> Vortex Flowmeter Transmitter Transfer Function/1

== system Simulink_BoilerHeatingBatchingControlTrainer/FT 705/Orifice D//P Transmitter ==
  In1 : Inport  RequirementInfo={} %GIDa_ea04ea7a_899b_4139_87bd_a0aa5a607789
  Bias : Bias  RequirementInfo={} %GIDa_57c2fa78_8f46_4824_91fd_664d3aea5689  Bias=4
  Orifice DP Flowmeter Transmitter Transfer Function : TransferFcn  RequirementInfo={} %GIDa_61370dfb_f0a9_46f7_a5c2_c2038d90759c  Numerator=[16]  Denominator=[2 1]
  Out1 : Outport  RequirementInfo={} %GIDa_321bd8b7_af77_44c1_9d36_567515e2a056
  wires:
  Bias/1 -> Out1/1
  Orifice DP Flowmeter Transmitter Transfer Function/1 -> Bias/1
  In1/1 -> Orifice DP Flowmeter Transmitter Transfer Function/1

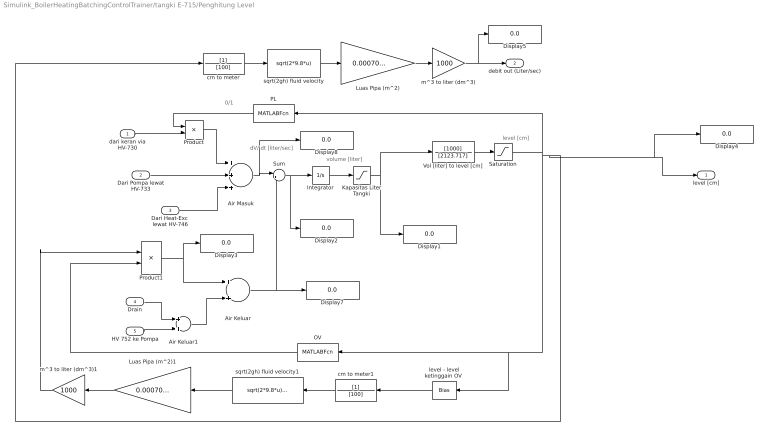
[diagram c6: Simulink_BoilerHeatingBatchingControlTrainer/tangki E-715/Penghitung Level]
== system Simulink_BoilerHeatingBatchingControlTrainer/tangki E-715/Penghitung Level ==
  note: 0/1
  note: dV/ dt [liter/sec]
  note: level [cm]
  note: volume [liter]
  dari keran via HV-730 : Inport  RequirementInfo={} %GIDa_d83a700a_7cab_4004_9a5d_fdfecec237f7
  Dari Pompa lewat HV-733 : Inport  RequirementInfo={} %GIDa_9a537d76_bde4_4273_90c4_02c6f5307bce  Port=2
  Dari Heat-Exc  lewat HV-746 : Inport  RequirementInfo={} %GIDa_d60d004d_f647_4259_a155_f975b758ff15  Port=3
  Drain : Inport  RequirementInfo={} %GIDa_a35a1899_7d91_4283_b472_a0a438fc953f  Port=4
  HV 752 ke Pompa : Inport  RequirementInfo={} %GIDa_bf32f437_b7ef_4725_8fd5_86d057d33ef2  Port=5
  Air Keluar : Sum  RequirementInfo={} %GIDa_0c522f95_7100_4807_9cc9_9301b09fba8f
  Air Keluar1 : Sum  RequirementInfo={} %GIDa_59b90af4_cbee_4cdc_a965_b2c45b6e2998
  Air Masuk : Sum  RequirementInfo={} %GIDa_ea552526_39fe_41c9_93e3_938c5b2a4261  Inputs=+++
  Display{1..5,7..8} (7 alike) : Display
  Integrator : Integrator  RequirementInfo={} %GIDa_6309caa5_67f3_4016_b1d2_7572912a21d1
  Kapasitas Liter Tangki : Saturate  RequirementInfo={} %GIDa_6d1a4914_2e79_4a7e_9709_82bd63d540f9  UpperLimit=120  LowerLimit=-99999999999999999999999999999999999999999999999999999999
  Luas Pipa (m^2) : Gain  RequirementInfo={} %GIDa_854e7fee_b5b6_4b96_8696_2ce9daa92837  Gain=0.000706858347
  Luas Pipa (m^2)1 : Gain  RequirementInfo={} %GIDa_ab7a824a_1247_48a8_a80d_346463c36851  Gain=0.000706858347
  OV : MATLABFcn  RequirementInfo={} %GIDa_1b058600_1bd2_4b7f_bc23_a53a14e3e558  MATLABFcn=OV
  PL : MATLABFcn  RequirementInfo={} %GIDa_b69f99d9_11a4_4873_b402_e1e28d0a9aa9  MATLABFcn=PL
  Product : Product  RequirementInfo={} %GIDa_c6354596_7705_4406_bfde_858e9fd19a7e
  Product1 : Product  RequirementInfo={} %GIDa_a5004d6e_bb3b_471b_abae_c517d8f7ab66
  Saturation : Saturate  RequirementInfo={} %GIDa_52267c6a_458c_450a_ac4c_87a818a77517  UpperLimit=65.5  LowerLimit=0
  Sum : Sum  RequirementInfo={} %GIDa_8d45d476_8853_40d7_b2ce_83fd6d42a90a  Inputs=|+-
  Vol [liter] to level [cm] : TransferFcn  RequirementInfo={} %GIDa_67fadcc3_e32e_45ef_92bf_8fdad950ba7f  Numerator=[1000]  Denominator=[2123.717]
  cm to meter : TransferFcn  RequirementInfo={} %GIDa_735bb47e_3034_4869_ab9b_f1a0421f91be  Denominator=[100]
  cm to meter1 : TransferFcn  RequirementInfo={} %GIDa_0a759192_ec2a_4f62_8d9e_644e7909b7ea  Denominator=[100]
  "level - level ketinggain OV " : Bias  RequirementInfo={} %GIDa_bb67a166_7956_443d_af38_9d10b8e6fa7d  Bias=-60
  m^3 to liter (dm^3) : Gain  RequirementInfo={} %GIDa_544e9fa6_bcf3_4c09_bea5_d547be29d49c  Gain=1000
  m^3 to liter (dm^3)1 : Gain  RequirementInfo={} %GIDa_1245c12a_2c96_4912_9c2e_e87fb4dfd22d  Gain=1000
  sqrt(2gh) fluid velocity : Fcn  RequirementInfo={} %GIDa_364b54df_e2f7_471c_8ed7_6a41d1481d77  Expr=sqrt(2*9.8*u)
  sqrt(2gh) fluid velocity1 : Fcn  RequirementInfo={} %GIDa_36797f0c_79df_4e5d_955b_f4cee5ab1c9c  Expr=sqrt(2*9.8*u)+0.00001
  level [cm] : Outport  RequirementInfo={} %GIDa_377b4651_73da_46a0_8503_cec5ac57bc49
  debit out (Liter/sec) : Outport  RequirementInfo={} %GIDa_768cab63_c415_4cea_9dc2_7fe9978759bb  Port=2
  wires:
  Vol [liter] to level [cm]/1 -> Saturation/1
  Integrator/1 -> Kapasitas Liter Tangki/1
  Sum/1 -> Integrator/1, Display2/1
  Air Masuk/1 -> Display8/1, Sum/1
  Dari Heat-Exc  lewat HV-746/1 -> Air Masuk/3
  Product/1 -> Air Masuk/1
  dari keran via HV-730/1 -> Product/2
  PL/1 -> Product/1
  m^3 to liter (dm^3)1/1 -> Product1/1
  OV/1 -> Product1/2
  Product1/1 -> Display3/1, Air Keluar/1
  Drain/1 -> Air Keluar1/1
  HV 752 ke Pompa/1 -> Air Keluar1/2
  Air Keluar1/1 -> Air Keluar/2
  Air Keluar/1 -> Display7/1, Sum/2
  m^3 to liter (dm^3)/1 -> Display5/1, debit out (Liter/sec)/1
  sqrt(2gh) fluid velocity/1 -> Luas Pipa (m^2)/1
  Luas Pipa (m^2)/1 -> m^3 to liter (dm^3)/1
  cm to meter/1 -> sqrt(2gh) fluid velocity/1
  cm to meter1/1 -> sqrt(2gh) fluid velocity1/1
  sqrt(2gh) fluid velocity1/1 -> Luas Pipa (m^2)1/1
  Luas Pipa (m^2)1/1 -> m^3 to liter (dm^3)1/1
  "level - level ketinggain OV "/1 -> cm to meter1/1
  Dari Pompa lewat HV-733/1 -> Air Masuk/2
  Kapasitas Liter Tangki/1 -> Vol [liter] to level [cm]/1, Display1/1
  Saturation/1 -> "level - level ketinggain OV "/1, OV/1, Display4/1, level [cm]/1, cm to meter/1, PL/1

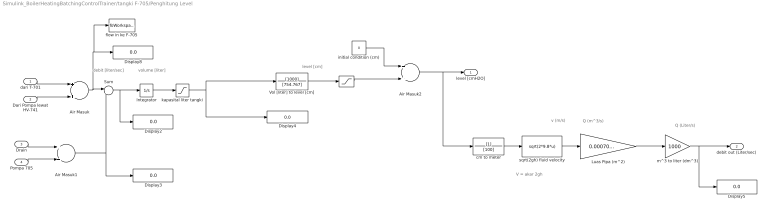
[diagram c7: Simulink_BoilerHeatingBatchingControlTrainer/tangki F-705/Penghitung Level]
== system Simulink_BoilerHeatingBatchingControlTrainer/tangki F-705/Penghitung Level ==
  note: V = akar 2gh
  note: Q (Liter/s)
  note: Q (m^3/s)
  note: v (m/s)
  note: debit [liter/sec]
  note: level [cm]
  note: volume [liter]
  dari T-701 : Inport  RequirementInfo={} %GIDa_b721c0c8_25bb_4028_a87c_6d7b9b4273c3
  Dari Pompa lewat HV-741 : Inport  RequirementInfo={} %GIDa_0d05a7b5_0e2a_4ba9_aa97_4beae1c0d14c  Port=2
  Drain : Inport  RequirementInfo={} %GIDa_d5e77f5b_792b_4b1f_8c8c_9ae8b6137790  Port=3
  Pompa 705 : Inport  RequirementInfo={} %GIDa_935b7ead_c867_4413_b131_9dd9333272c2  Port=4
  . : Saturate  RequirementInfo={} %GIDa_6c281582_efc2_487c_bffd_91d3676bb990  UpperLimit=119.5  LowerLimit=-999999999999999999999999999999999999999999999999999  LinearizeAsGain=off  ZeroCross=off
  Air Masuk : Sum  RequirementInfo={} %GIDa_ccac27af_5856_4cbf_9588_de6efc053c44
  Air Masuk1 : Sum  RequirementInfo={} %GIDa_b57b9f1a_1068_4822_8057_be9db6d61278
  Air Masuk2 : Sum  RequirementInfo={} %GIDa_2f458e0d_34ee_4831_850d_2c14d0d50bae
  Display{2..5,8} (5 alike) : Display
  Integrator : Integrator  RequirementInfo={} %GIDa_97bb95d7_59d0_48e5_97e1_cafbb3e674ba
  Luas Pipa (m^2) : Gain  RequirementInfo={} %GIDa_d5f293a5_dee0_48be_9cb1_c29654f86bb9  Gain=0.000706858347
  Sum : Sum  RequirementInfo={} %GIDa_06115cfb_965a_4117_b6e2_9d6ee1761ded  Inputs=|+-
  Vol [liter] to level [cm] : TransferFcn  RequirementInfo={} %GIDa_9157dd10_86b3_4991_9260_c05f22c268a1  Numerator=[1000]  Denominator=[754.767]
  cm to meter : TransferFcn  RequirementInfo={} %GIDa_ab32d74a_a7ce_4e58_ace4_9522443d9ab7  Denominator=[100]
  "flow in ke F-705 " : ToWorkspace  VariableName=flow_in  SampleTime=-1
  "initial condition (cm) " : Constant  Value=0
  kapasital liter tangki : Saturate  RequirementInfo={} %GIDa_429f95f8_af51_406b_bae6_8e8d4c9db921  UpperLimit=100  LowerLimit=-99999999999999999999999999999999999999999999999999  LinearizeAsGain=off  ZeroCross=off
  m^3 to liter (dm^3) : Gain  RequirementInfo={} %GIDa_1a89ef4f_4541_4ebe_9fb0_95a7020f2097  Gain=1000
  sqrt(2gh) fluid velocity : Fcn  RequirementInfo={} %GIDa_783557ad_37e8_4f53_9b57_037cd56e5f88  Expr=sqrt(2*9.8*u)
  level [cmH2O] : Outport  RequirementInfo="{'linktype_rmi_simulink' 'D' ':376' 'true' 'D/Lamp  (SubSystem)' '' } %GIDa_3dde4e03_dc02_4e80_b2bc_bc84ddf2d094"
  debit out (Liter/sec) : Outport  RequirementInfo={} %GIDa_3eef054a_9faa_437a_942b_cf8add6bfe79  Port=2
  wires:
  Sum/1 -> Display2/1, Integrator/1
  Air Masuk/1 -> Sum/1, "flow in ke F-705 "/1, Display8/1
  Dari Pompa lewat HV-741/1 -> Air Masuk/2
  dari T-701/1 -> Air Masuk/1
  Integrator/1 -> kapasital liter tangki/1
  Drain/1 -> Air Masuk1/1
  Air Masuk1/1 -> Sum/2, Display3/1
  sqrt(2gh) fluid velocity/1 -> Luas Pipa (m^2)/1
  Luas Pipa (m^2)/1 -> m^3 to liter (dm^3)/1
  Pompa 705/1 -> Air Masuk1/2
  cm to meter/1 -> sqrt(2gh) fluid velocity/1
  kapasital liter tangki/1 -> Vol [liter] to level [cm]/1, Display4/1
  Vol [liter] to level [cm]/1 -> ./1
  m^3 to liter (dm^3)/1 -> Display5/1, debit out (Liter/sec)/1
  ./1 -> Air Masuk2/2
  Air Masuk2/1 -> cm to meter/1, level [cmH2O]/1
  "initial condition (cm) "/1 -> Air Masuk2/1

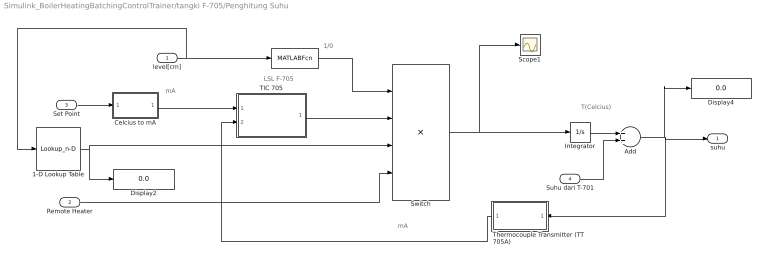
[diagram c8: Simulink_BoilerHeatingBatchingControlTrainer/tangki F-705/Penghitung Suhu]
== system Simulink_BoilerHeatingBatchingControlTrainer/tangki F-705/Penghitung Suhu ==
  note: mA
  note: mA
  note: T(Celcius)
  note: LSL F-705
  note: 1/0
  level[cm] : Inport  RequirementInfo={} %GIDa_af478511_908b_4604_bfd3_b01a4b9af0ed
  Remote Heater : Inport  RequirementInfo={} %GIDa_00e1230e_6914_4335_8fef_c71b0855354d  Port=2
  Set Point : Inport  RequirementInfo={} %GIDa_0dee31ff_83ad_44bf_81c7_3fb3ae19355c  Port=3
  Suhu dari T-701 : Inport  Port=4
  " " : MATLABFcn  RequirementInfo="{'linktype_rmi_simulink' 'D' ':376' 'true' 'D/Lamp  (SubSystem)' '' } %GIDa_2ad5c819_4590_4a52_bffc_872927469afa"  MATLABFcn=LSL705
  1-D Lookup Table : Lookup_n-D  NumberOfTableDimensions=1  BreakpointsForDimension1=[20,30,40,50]  Table=[0.1204,0.08678,0.06899,0.05397]  InternalRulePriority=Speed  RndMeth=Simplest
  Add : Sum
  Celcius to mA : Subsystem  RequirementInfo={} %GIDa_a308ac00_69ff_4bbc_855b_8e264b0f0d31
  Display2 : Display
  Display4 : Display
  Integrator : Integrator  RequirementInfo={} %GIDa_3341c1cb_0aca_4615_b1d8_bd3985964488
  Scope1 : Scope
  Switch : Product  RequirementInfo={} %GIDa_9bb206da_9dce_4a1b_ad00_3801d807c1ae  Inputs=4
  TIC 705 : Subsystem  RequirementInfo={} %GIDa_5a79bba3_b1e1_479d_91b9_40de190a25a2
  Thermocouple Transmitter (TT 705A) : Subsystem  RequirementInfo={} %GIDa_5459d06b_300c_4efe_b66c_83d7be41133f
  suhu : Outport  RequirementInfo={} %GIDa_6e4df8d2_5595_4382_a207_d16b04290d93
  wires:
  level[cm]/1 -> 1-D Lookup Table/1, " "/1
  Switch/1 -> Scope1/1, Integrator/1
  Remote Heater/1 -> Switch/4
  TIC 705/1(Out1) -> Switch/2
  " "/1 -> Switch/1
  1-D Lookup Table/1 -> Display2/1, Switch/3
  Thermocouple Transmitter (TT 705A)/1(Out2) -> TIC 705/2(In3)
  Set Point/1 -> Celcius to mA/1(In1)
  Celcius to mA/1(Out1) -> TIC 705/1(In2)
  Integrator/1 -> Add/1
  Add/1 -> Display4/1, Thermocouple Transmitter (TT 705A)/1(In2), suhu/1
  Suhu dari T-701/1 -> Add/2

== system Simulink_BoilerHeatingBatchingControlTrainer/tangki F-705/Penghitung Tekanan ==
  Suhu : Inport  RequirementInfo={} %GIDa_7c27ca46_27a2_4e81_849b_0f88d8bcecec
  Level : Inport  RequirementInfo={} %GIDa_7e7114e7_19a3_48cf_ae5b_5723ad3cad4e  Port=2
  Bourdon Tube : Lookup_n-D  RequirementInfo={} %GIDa_575231b5_4d22_4fad_a392_d95fddd33a5e  BreakpointsForDimension1=[28,29,30,31,32,33,34,35,36,37,38,39,40,41,42,43,44,45,46,47,48,49,50,51,52,53,54,55,56,57,58,59,60,61,62,63,64,65,66,67,68,69,70,71,72,73,74,75,76,77,78,79,80,81,82,83,84,85,86,87,88,89,90,91,92,93,94,95,96,97,98,99,100]  BreakpointsForDimension2=[30,40,50]  Table=reshape([0,0,0,0,0,0,0,0,0,0,0,0,0,0,0,0,0,0,0,0,0,0,0,0,0,0,0,0,0,0,0,0,0,0,0,0,0,0,0,0,0,0,0,0,0,0,0,0,1,3,9,10,10,11,12,13,14,14,15,15,16,18,20,20,22,24,25,26,27,28,29,29,30,0,0,0,0,0,0,0,0,0,0,0,0,0,0,0,0,0,0,0,0,0,0,0,0,0,0,0,0,0,0,0,0,0,0,0,0,0,0,0,0,0,0,0,0,0,0,1,5,8,7,10,10,11,12,13,14,14,15,16,17,18,20,21,22,24,25,25,27,29,30,31,31,32,0,0,0,0,0,0,0,0,0,0,0,0,0,0,0,0,0,0,0,0,0,0,0,0,0,0,0,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  InternalRulePriority=Speed  RndMeth=Simplest
  Display1 : Display
  Pressure tangki (mbar) : Outport  RequirementInfo={} %GIDa_a354c4c3_231b_4c75_be7e_18002176496b
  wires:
  Suhu/1 -> Bourdon Tube/1
  Level/1 -> Bourdon Tube/2
  Bourdon Tube/1 -> Display1/1, Pressure tangki (mbar)/1
